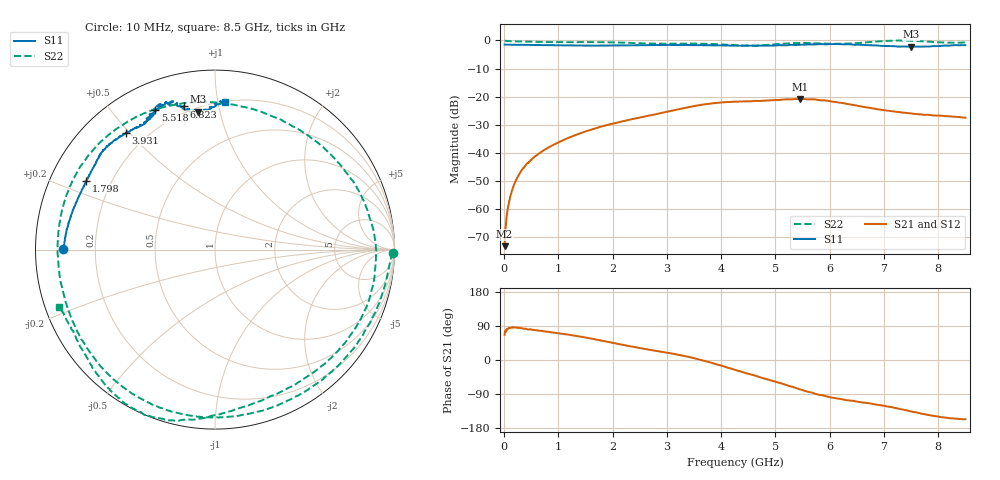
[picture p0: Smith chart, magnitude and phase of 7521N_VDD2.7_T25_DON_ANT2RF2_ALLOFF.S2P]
!Agilent Technologies,E5071C,MY46417908,A.11.23
!Date: Thu Jul 30 15:14:07 2020
!Data & Calibration Information:
!Freq	S11:SOLT2(ON)	S21:SOLT2(ON)	S12:SOLT2(ON)	S22:SOLT2(ON)
!PortZ  Port1:50+j0  Port2:50+j0
!Above PortZ is port z conversion or system Z0 setting when saving the data.
!When reading, reference impedance value at option line is always used.
# Hz S dB R 50
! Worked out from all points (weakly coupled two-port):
!   1601 points, 10 MHz to 8.5 GHz, reference 50 ohm
!   highest |S21| = -20.80 dB at 5.46 GHz (marker M1); lowest = -73.2 dB at 10 MHz (marker M2)
!   lowest |S11| = -2.2 dB at 7.497 GHz (marker M3), VSWR 7.86, Z = 11.2 + j43.1 ohm
!   |S11| at or under -10 dB: nowhere
!   |S22| runs from -1.9 to 0.0 dB; largest |S21 - S12| = 0.00077
!   S11 on the Smith chart (normalised r, x): 10 MHz: 0.08, +0.00; 1.798 GHz: 0.11, +0.25; 3.931 GHz: 0.12, +0.49; 5.518 GHz: 0.12, +0.65; 6.823 GHz: 0.17, +0.79; 8.5 GHz: 0.20, +1.05
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1e7  -1.46 179.9  -73.24 66.4  -74.16 77.0  -0.06 -1.0
6.836875e7  -1.50 178.9  -59.89 81.6  -59.94 82.5  -0.21 -5.1
1.214312e8  -1.50 178.0  -55.03 84.6  -55.05 85.4  -0.26 -8.5
3.28375e8  -1.54 175.1  -46.10 84.0  -46.03 83.8  -0.37 -21.6
8.749188e8  -1.68 166.7  -37.51 73.0  -37.51 73.1  -0.57 -54.4
1.426769e9  -1.79 157.9  -32.89 61.2  -32.90 61.1  -0.58 -85.7
1.798206e9  -1.80 151.8  -30.63 51.1  -30.63 51.1  -0.60 -106.7
2.328831e9  -1.73 144.8  -28.14 36.1  -28.14 36.1  -0.86 -137.3
2.843538e9  -1.60 140.0  -26.04 23.1  -26.04 23.1  -1.13 -166.8
3.432531e9  -1.62 134.3  -23.62 7.2  -23.62 7.2  -1.10 157.6
3.931319e9  -1.74 127.3  -22.19 -12.1  -22.18 -12.1  -1.31 120.8
4.255e9  -1.82 123.4  -21.77 -26.0  -21.79 -25.9  -1.69 92.9
4.621131e9  -1.90 120.3  -21.54 -41.3  -21.51 -41.2  -1.81 59.9
4.987262e9  -1.80 116.9  -21.20 -57.1  -21.17 -57.1  -1.38 27.9
5.459519e9  -1.54 113.4  -20.80 -77.8  -20.81 -78.0  -0.89 -11.6
5.517888e9  -1.47 113.2  -20.85 -80.3  -20.84 -80.3  -0.90 -16.4
5.671769e9  -1.43 113.5  -20.93 -86.0  -20.91 -86.0  -0.95 -28.7
6.128106e9  -1.30 108.2  -21.97 -101.3  -21.96 -101.4  -1.19 -61.9
6.823225e9  -1.76 102.4  -24.27 -117.0  -24.23 -117.1  -0.42 -96.6
7.088538e9  -1.97 100.5  -25.04 -123.3  -25.04 -123.4  -0.11 -106.3
7.497119e9  -2.22 96.9  -25.99 -135.8  -25.93 -135.5  -0.08 -121.6
8.5e9  -1.66 86.1  -27.48 -156.3  -27.56 -156.9  -0.68 -159.6
